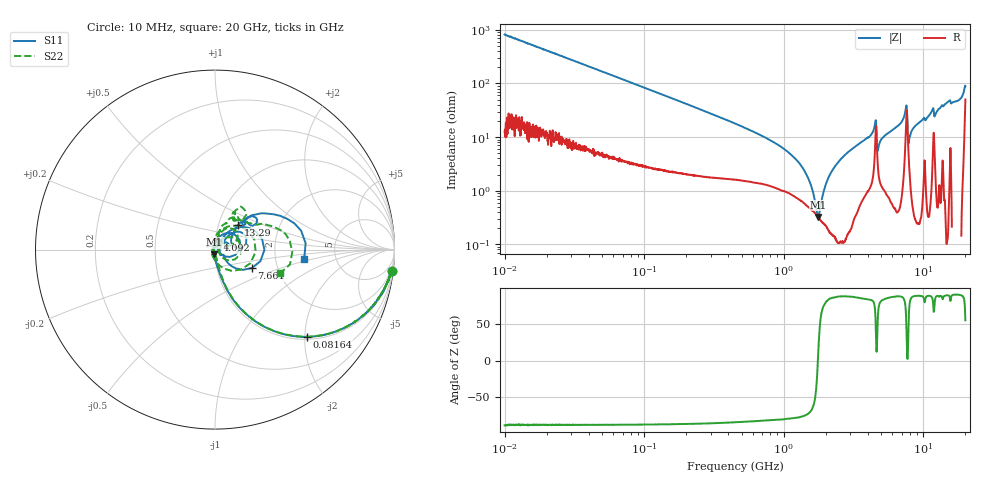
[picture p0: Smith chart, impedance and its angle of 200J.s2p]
!Keysight Technologies,P5008B,MY61100088,A.16.20.02
!Date: Monday, November 06, 2023 16:36:15
!Correction: S11(C  2-Port  )
!S21(C  2-Port  )
!S12(C  2-Port  )
!S22(C  2-Port  )
!S2P File: Measurements: S11, S21, S12, S22:Log Frequency Sweep
# Hz S  dB  R 50
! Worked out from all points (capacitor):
!   1601 points, 10 MHz to 20 GHz, reference 50 ohm
!   read as one part in series: C = 19.4 pF near 10.39 MHz
!   lowest |Z| = 324 mohm at 1.757 GHz (marker M1)
!   series resonance near 1.755 GHz, so ESL is about 420 pH
!   S11 on the Smith chart (normalised r, x): 10 MHz: 1, -16; 81.64 MHz: 1.06, -2.06; 4.092 GHz: 1.01, +0.10; 7.661 GHz: 1.47, -0.32; 13.29 GHz: 1.24, +0.36; 20 GHz: 2.93, -0.41
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1e7  -0.08 -6.9  -18.38 82.2  -18.38 82.2  -0.08 -6.9
3.555162e7  -0.80 -22.8  -8.24 65.6  -8.24 65.6  -0.81 -22.8
8.164123e7  -3.01 -43.4  -3.27 44.7  -3.28 44.7  -3.04 -43.4
1.263918e8  -5.25 -55.1  -1.73 32.8  -1.74 32.8  -5.31 -55.1
4.472136e8  -14.65 -75.9  -0.29 9.7  -0.29 9.7  -15.28 -75.3
1.589917e9  -29.02 -94.1  -0.09 -0.4  -0.09 -0.4  -33.72 -92.9
1.756711e9  -31.68 -97.5  -0.08 -1.2  -0.08 -1.2  -37.00 -103.1
2.39224e9  -45.23 -177.3  -0.07 -3.6  -0.08 -3.6  -42.83 168.8
3.019248e9  -32.19 110.3  -0.09 -5.7  -0.10 -5.7  -39.73 101.1
4.092041e9  -25.64 79.4  -0.13 -9.0  -0.13 -9.0  -29.08 58.2
4.4999e9  -19.01 54.6  -0.52 -12.9  -0.52 -12.9  -19.43 40.5
4.924959e9  -35.44 39.8  -0.11 -8.9  -0.11 -9.0  -33.49 23.2
5.652411e9  -29.98 64.2  -0.06 -11.8  -0.07 -11.8  -27.26 67.5
6.738606e9  -23.47 57.1  -0.08 -15.9  -0.08 -15.9  -22.56 85.8
7.410252e9  -14.76 42.8  -0.68 -22.6  -0.68 -22.6  -15.65 53.8
7.660815e9  -12.79 -26.8  -1.88 -9.1  -1.89 -9.1  -14.83 -38.2
8.110221e9  -29.42 -37.0  -0.10 -14.3  -0.10 -14.3  -33.34 -134.7
8.424378e9  -31.82 2.6  -0.04 -16.3  -0.04 -16.3  -36.48 154.7
1.141771e10  -18.26 45.0  -0.12 -27.8  -0.12 -27.8  -18.60 66.7
1.329228e10  -14.43 46.7  -0.18 -31.4  -0.18 -31.4  -14.71 65.6
1.818725e10  -12.57 44.9  -0.29 -48.4  -0.29 -48.4  -12.89 43.5
2e10  -6.02 -6.0  -4.42 -53.4  -4.42 -53.4  -8.27 -20.1
